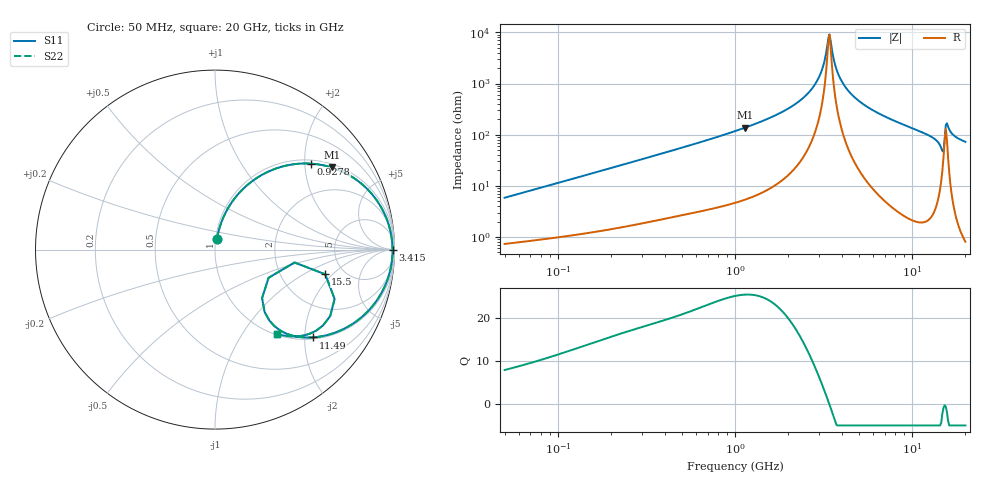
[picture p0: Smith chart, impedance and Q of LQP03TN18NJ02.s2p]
!Murata Part Number: LQP03TN18NJ02
!These Parameters are Measured in Series Mode Connection
!  o--[Z]--o
!Port1  Port2
!  o-------o
!Freq. Start=50[MHz] Stop=20[GHz], 401[Steps]
# Hz S RI R 50
!Freq.(Hz) S11(Real) S11(Imag) S21(Real) S21(Imag) S12(Real) S12(Imag) S22(Real) S22(Imag)
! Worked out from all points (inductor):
!   401 points, 50 MHz to 20 GHz, reference 50 ohm
!   read as one part in series: L = 18.3 nH near 51.52 MHz
!   highest Q = 25.5 at 1.144 GHz (marker M1), where L = 19.2 nH
!   self-resonance near 3.364 GHz
!   S11 on the Smith chart (normalised r, x): 50 MHz: 1.01, +0.12; 927.8 MHz: 1.09, +2.15; 3.415 GHz: open; 11.49 GHz: 1.04, -2.20; 15.5 GHz: 3.60, -1.64; 20 GHz: 1.02, -1.45
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5e7  0.0106 0.0571  0.9894 -0.0571  0.9894 -0.0571  0.0106 0.0571
1.364002e8  0.0337 0.1469  0.9663 -0.1469  0.9663 -0.1469  0.0337 0.1469
3.721004e8  0.1583 0.3398  0.8417 -0.3398  0.8417 -0.3398  0.1583 0.3398
9.278425e8  0.535 0.4791  0.465 -0.4791  0.465 -0.4791  0.535 0.4791
1e9  0.5761 0.4747  0.4239 -0.4747  0.4239 -0.4747  0.5761 0.4747
1.144317e9  0.6501 0.4577  0.3499 -0.4577  0.3499 -0.4577  0.6501 0.4577
1.962148e9  0.8958 0.282  0.1042 -0.282  0.1042 -0.282  0.8958 0.282
2.728004e9  0.9733 0.119  0.0267 -0.119  0.0267 -0.119  0.9733 0.119
3.075291e9  0.9855 0.0553  0.0145 -0.0553  0.0145 -0.0553  0.9855 0.0553
3.314454e9  0.9888 0.015  0.0112 -0.015  0.0112 -0.015  0.9888 0.015
3.415248e9  0.9892 -0.00121  0.0108 0.00121  0.0108 0.00121  0.9892 -0.00121
3.792786e9  0.9862 -0.0579  0.0138 0.0579  0.0138 0.0579  0.9862 -0.0579
4.275624e9  0.9746 -0.1223  0.0254 0.1223  0.0254 0.1223  0.9746 -0.1223
5.352748e9  0.929 -0.2388  0.071 0.2388  0.071 0.2388  0.929 -0.2388
7.442007e9  0.8052 -0.3861  0.1948 0.3861  0.1948 0.3861  0.8052 -0.3861
1.149051e10  0.5461 -0.4892  0.4539 0.4892  0.4539 0.4892  0.5461 -0.4892
1.354865e10  0.396 -0.4672  0.604 0.4672  0.604 0.4672  0.396 -0.4672
1.460232e10  0.2764 -0.3475  0.7236 0.3475  0.7236 0.3475  0.2764 -0.3475
1.550395e10  0.6143 -0.1376  0.3857 0.1376  0.3857 0.1376  0.6143 -0.1376
1.597544e10  0.642 -0.3701  0.358 0.3701  0.358 0.3701  0.642 -0.3701
1.670968e10  0.5323 -0.4669  0.4677 0.4669  0.4677 0.4669  0.5323 -0.4669
2e10  0.3464 -0.4703  0.6536 0.4703  0.6536 0.4703  0.3464 -0.4703
